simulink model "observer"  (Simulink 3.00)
settings: Solver=ode45  StartTime=0.0  StopTime=10.0  RelTol=1e-3
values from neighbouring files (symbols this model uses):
  A = [0 1 0 0;0 0 -mb*g/(1-mb) 0;0 0 0 1;0 0 m2_bar*g/(1-mb) 0]    [EXP7_1.M]    (also in EXP6_10.M = [0 1 0;0 -1.799 6.953;0 0.939 -1.660]; EXP6_8.M = [a11 a12 0 -g;a21 a22 1 0;a31 a31 a33 0;0 1 0 0]; EXP6_9.m = [a11 a12 0 -g;a21 a22 1 0;a31 a31 a33 0;0 1 0 0]; EXP7_2.M)
  B = [0;1/((m+M)*(1-mb));0;-m2_bar/((m+M)*(1-mb))]    [EXP7_1.M]    (also in EXP6_10.M = [0 0;-28.97 -6.453;-0.174 -0.230]; EXP6_8.M = [b1;b2;b3;0]; EXP6_9.m = [b1;b2;b3;0]; EXP7_2.M)
  C = [1 0 0 0]    [EXP7_1.M]    (also in EXP6_8.M; EXP6_9.m; EXP7_2.M = [1 0 0 0;0 0 1 0]; EXP7_21.m = [1 0 0 0;0 0 1 0])
  L = L_ext'    [EXP7_1.M]    (also in EXP5_3.M = 0.35; ODE.M = par_in(5); EXP7_2.M = [-10 1 0 0;0 0 -10 1]; EXP7_21.m = [-10 1 0 0;0 0 -10 1])
libraries: simulink3 x7

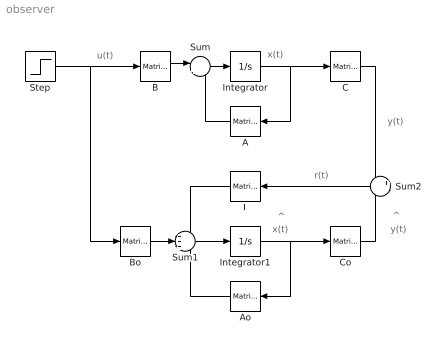
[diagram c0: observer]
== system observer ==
  note: u(t)
  note: x(t)
  note: r(t)
  note: y(t)
  note: y(t)
  note: ^
  note: x(t)
  note: ^
  A : simulink3/Math/Matrix Gain  Orientation=left  K=A
  Ao : simulink3/Math/Matrix Gain  Orientation=left  K=A
  B : simulink3/Math/Matrix Gain  K=B
  Bo : simulink3/Math/Matrix Gain  K=B
  C : simulink3/Math/Matrix Gain  K=C
  Co : simulink3/Math/Matrix Gain  K=C
  Integrator : Integrator  ExternalReset=none  InitialConditionSource=internal  InitialCondition=[0.2 .1 -0.5 5]  LimitOutput=off  UpperSaturationLimit=inf  LowerSaturationLimit=-inf  ShowSaturationPort=off  ShowStatePort=off  AbsoluteTolerance=auto
  Integrator1 : Integrator  ExternalReset=none  InitialConditionSource=internal  InitialCondition=0  LimitOutput=off  UpperSaturationLimit=inf  LowerSaturationLimit=-inf  ShowSaturationPort=off  ShowStatePort=off  AbsoluteTolerance=auto
  L : simulink3/Math/Matrix Gain  Orientation=left  K=L
  Step : Step  Time=0  Before=0  After=1  SampleTime=0
  Sum : Sum  Inputs=|++  SaturateOnIntegerOverflow=on
  Sum1 : Sum  Inputs=+++  SaturateOnIntegerOverflow=on
  Sum2 : Sum  Orientation=left  Inputs=+-  SaturateOnIntegerOverflow=on
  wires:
  B/1 -> Sum/1
  Sum/1 -> Integrator/1
  Integrator/1 -> C/1, A/1
  Sum1/1 -> Integrator1/1
  Step/1 -> B/1, Bo/1
  C/1 -> Sum2/1
  Co/1 -> Sum2/2
  Bo/1 -> Sum1/2
  Integrator1/1 -> Co/1, Ao/1
  L/1 -> Sum1/1
  A/1 -> Sum/2
  Ao/1 -> Sum1/3
  Sum2/1 -> L/1
